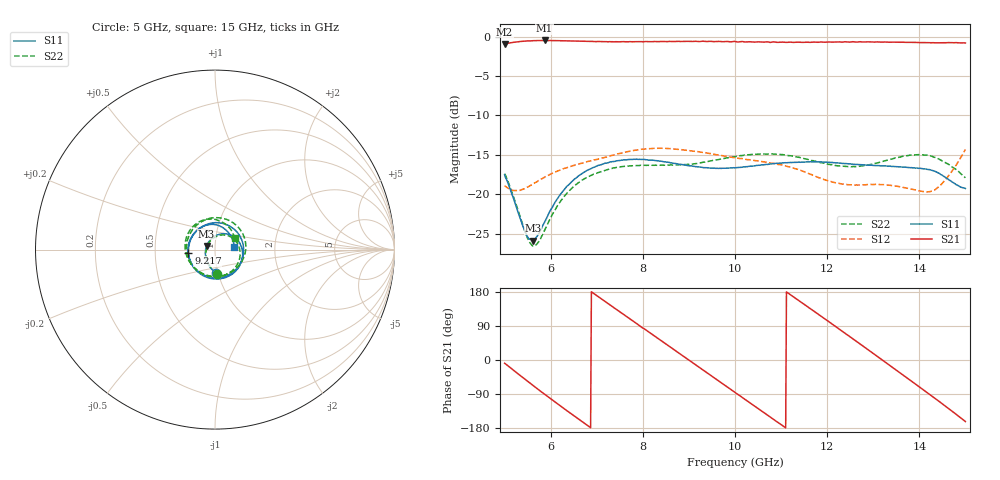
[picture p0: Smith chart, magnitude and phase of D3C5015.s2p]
! 4/14/2021 1:34:34 PM
! C:\USERS\DITOM\DESKTOP\SINGLE JUNCTION ISOLATOR DATA\5.0 -15.0 GHZ (D3I5015).S2P
! CHANNEL.1
! TR.MEASUREMENT
! CORRECTED.DATA
# GHZ S RI R 50.0
! FREQ.GHZ  S11RE  S11IM  S21RE  S21IM  S12RE  S12IM  S22RE  S22IM
!; PortSelection: Port_12
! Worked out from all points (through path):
!   601 points, 5 GHz to 15 GHz, reference 50 ohm
!   highest |S21| = -0.50 dB at 5.867 GHz (marker M1); lowest = -0.9 dB at 5 GHz (marker M2)
!   lowest |S11| = -25.9 dB at 5.617 GHz (marker M3), VSWR 1.11, Z = 45.5 + j1.81 ohm
!   |S11| at or under -10 dB: start of sweep to end of sweep
!   |S22| runs from -26.6 to -14.9 dB; largest |S21 - S12| = 0.86
!   S11 on the Smith chart (normalised r, x): 5 GHz: 0.98, -0.26; 9.217 GHz: 0.74, -0.03; 15 GHz: 1.24, +0.04
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5  0.00708 -0.1327  0.8876 -0.134  0.0275 -0.11  0.011 -0.1348
5.616667  -0.0469 0.0199  0.3631 -0.8685  -0.0177 -0.115  -0.0456 0.0115
5.866667  -0.016 0.0645  -0.006 -0.9444  -0.054 -0.1166  -0.0187 0.056
6.666667  0.1218 0.0572  -0.8848 -0.2979  -0.1571 -0.00789  0.1088 0.0554
7.116667  0.1539 -0.019  -0.8703 0.32  -0.1407 0.0952  0.1395 -0.0119
7.616667  0.1239 -0.1095  -0.4238 0.8231  -0.042 0.1804  0.1132 -0.0993
8.35  -0.0195 -0.1616  0.5309 0.7614  0.1578 0.1161  -0.0291 -0.1504
8.8  -0.1097 -0.1094  0.8918 0.2674  0.1916 -0.0164  -0.1212 -0.0948
9.216667  -0.1481 -0.0181  0.88 -0.2981  0.1379 -0.1244  -0.1579 0.00063
10  -0.0612 0.1341  0.0725 -0.9281  -0.0581 -0.1607  -0.0654 0.16
10.43333  0.0361 0.1473  -0.4926 -0.7798  -0.1372 -0.0888  0.038 0.1752
10.88333  0.1242 0.0963  -0.8699 -0.3032  -0.1551 0.017  0.1327 0.1214
11.26667  0.1585 0.0144  -0.8941 0.2088  -0.113 0.0937  0.1709 0.0348
11.66667  0.1405 -0.0777  -0.6261 0.6754  -0.038 0.1277  0.1514 -0.0622
12.05  0.0718 -0.1423  -0.1575 0.9106  0.0266 0.1182  0.0838 -0.1301
12.41667  -0.0178 -0.1556  0.3456 0.8581  0.0729 0.0896  -0.00713 -0.1501
12.91667  -0.1201 -0.0949  0.8404 0.3841  0.1122 0.0272  -0.1202 -0.0962
13.35  -0.1508 -0.00011  0.8951 -0.213  0.1065 -0.0412  -0.1655 0.00217
13.8  -0.1153 0.0919  0.5509 -0.7355  0.0611 -0.0898  -0.1377 0.1114
14.18333  -0.0422 0.1374  0.0429 -0.9125  0.0196 -0.1017  -0.0581 0.1671
14.56667  0.0513 0.117  -0.4805 -0.7767  -0.0149 -0.1231  0.0391 0.1539
15  0.1076 0.0169  -0.867 -0.2754  -0.1227 -0.148  0.1113 0.062
